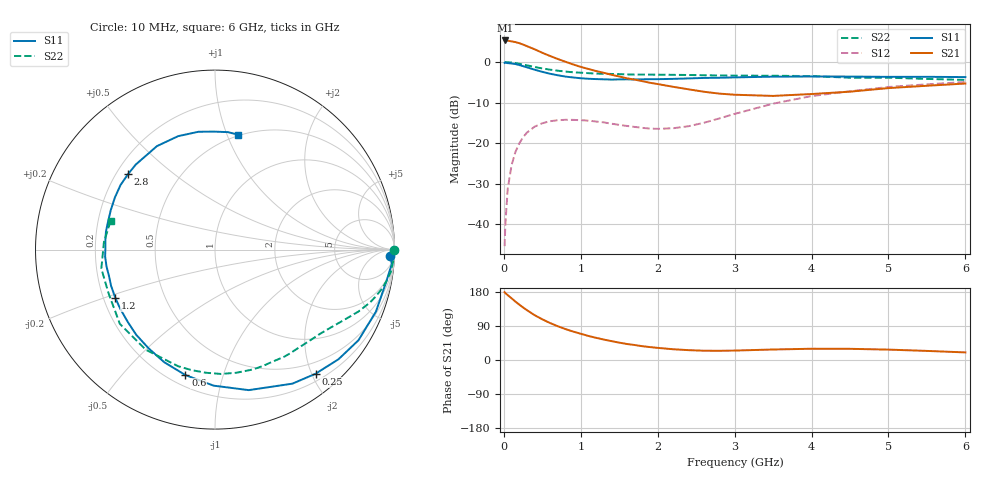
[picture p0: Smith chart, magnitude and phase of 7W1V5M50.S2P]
! Infineon Technologies  Discrete & RF Semiconductors
! BFS17W
! Si NPN RF Bipolar Junction Transistor in SOT323
! VCE = 1.5 V  IC = 0.5 mA
! Common Emitter S-Parameters:  August  1999
# GHz  S  MA  R  50
!  f  S11  S21  S12  S22
! GHz  MAG  ANG  MAG  ANG  MAG  ANG  MAG  ANG
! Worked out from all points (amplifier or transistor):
!   36 points, 10 MHz to 6 GHz, reference 50 ohm
!   highest |S21| = 5.3 dB at 20 MHz (marker M1)
!   |S21| within 3 dB of that: start of sweep to 495.5 MHz
!   unconditionally stable (mu >= 1): 1.138 GHz to end of sweep
!   at 250 MHz: K = 0.24, MSG = 11.4 dB, |S12| = -18.5 dB
!   at 1.4 GHz: K = 1.22, MAG = 3.2 dB, |S12| = -15.2 dB
!   at 6 GHz: K = 1.12, MAG = -2.3 dB, |S12| = -4.9 dB
!   S11 on the Smith chart (normalised r, x): 10 MHz: 26, -40; 250 MHz: 0.31, -2.06; 600 MHz: 0.26, -0.76; 1.2 GHz: 0.25, -0.22; 2.8 GHz: 0.25, +0.35; 6 GHz: 0.49, +1.10
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0.01  0.9775 -2.0  1.833 179.1  0.0054 86.8  0.9999 -0.2
0.02  0.9881 -4.6  1.846 176.6  0.0101 85.2  0.9959 -1.4
0.05  0.9709 -10.6  1.836 171.3  0.0273 83.6  0.9949 -3.6
0.1  0.9609 -21.1  1.797 162.9  0.0535 76.9  0.9875 -7.2
0.15  0.9455 -32.3  1.762 154.2  0.0779 70.3  0.971 -10.5
0.25  0.8901 -51.0  1.643 138.6  0.1185 58.7  0.9313 -16.4
0.3  0.8625 -60.0  1.57 131.5  0.1352 54.1  0.9124 -18.9
0.4  0.8052 -76.5  1.438 118.3  0.1601 45.1  0.87 -23.4
0.5  0.758 -90.6  1.301 107.4  0.1763 38.1  0.8344 -26.9
0.6  0.7181 -103.3  1.189 97.6  0.1868 32.4  0.8062 -30.1
0.8  0.6627 -124.0  1.01 81.7  0.1946 24.3  0.7642 -36.1
1.1  0.6225 -147.9  0.822 63.4  0.1899 17.3  0.7296 -44.7
1.2  0.6173 -154.0  0.775 58.5  0.1851 16.1  0.722 -47.8
1.6  0.6134 -176.5  0.631 42.2  0.1634 17.0  0.7049 -60.3
2.2  0.6211 159.2  0.496 28.4  0.153 35.4  0.6964 -80.4
2.8  0.6414 139.1  0.409 24.3  0.202 52.7  0.684 -101.2
3.5  0.6611 119.3  0.383 27.7  0.3073 54.6  0.6782 -124.6
4  0.6646 108.0  0.404 29.7  0.3813 49.4  0.6726 -142.0
4.5  0.663 98.0  0.432 29.5  0.4371 43.0  0.6412 -157.6
5  0.6573 90.4  0.478 27.4  0.4936 36.7  0.6421 -170.5
5.5  0.6584 83.8  0.511 24.0  0.5322 30.5  0.6202 176.1
6  0.653 78.5  0.544 20.0  0.5682 24.7  0.603 164.5
